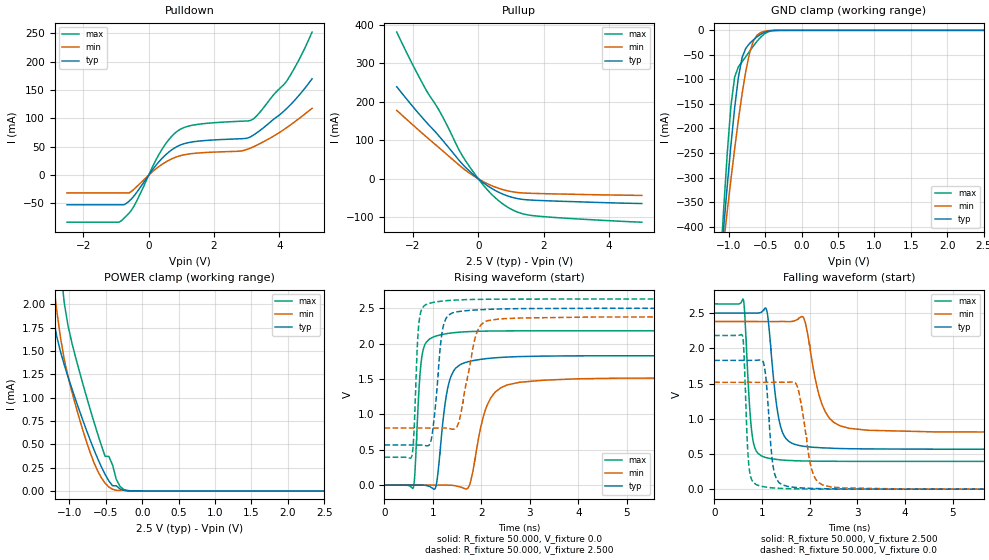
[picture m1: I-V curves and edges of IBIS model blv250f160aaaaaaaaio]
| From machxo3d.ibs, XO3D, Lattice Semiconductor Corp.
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|   Model blv250f160aaaaaaaaio
[Model] blv250f160aaaaaaaaio
Model_type I/O
Polarity   Non-Inverting
Enable   Active-Low
Vinl =  1.150V
Vinh =  1.350V
Vmeas =  1.250V
Cref =  3.000pF
Rref =  50.000
Vref =  1.250V
C_comp   4.200pF   3.800pF   7.500pF
[Temperature Range]   25.000   0.105k   -40.000
[Voltage Range]   2.500V   2.380V   2.630V
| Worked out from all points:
|   slope of the pulldown table from 0 to 0.375 V, typ, clamps not added: 13.6 ohm
|   slope of the pullup table from 0 to 0.375 V, typ, clamps not added: 16.3 ohm
|   GND clamp passes 1 mA (typ) near -0.43 V on its own axis
|   POWER clamp passes 1 mA (typ) near -0.92 V on its own axis
|   rising waveform, R_fixture 50.000, V_fixture 0.0: 20-80 % time 206ps typ, 326ps min, 111ps max; typ from 0 V to 1.83 V
|   rising waveform, R_fixture 50.000, V_fixture 2.500: 20-80 % time 152ps typ, 261ps min, 82.5ps max; typ from 0.567 V to 2.5 V
|   falling waveform, R_fixture 50.000, V_fixture 2.500: 20-80 % time 196ps typ, 321ps min, 119ps max; typ from 2.5 V to 0.567 V
|   falling waveform, R_fixture 50.000, V_fixture 0.0: 20-80 % time 127ps typ, 212ps min, 78.8ps max; typ from 1.83 V to 0 V
[Pulldown]
|Voltage   I(typ)   I(min)   I(max)
-2.5V     -52.31mA   -31.26mA   -82.98mA
-828mV    -52.31mA   -31.26mA   -79.94mA
-600mV    -45.86mA   -31.26mA   -66.93mA
-448mV    -36.56mA   -24.66mA   -54.4mA
160mV     12.89mA    8.306mA    19.88mA
464mV     32.88mA    21.18mA    50.69mA
996mV     53.81mA    34.73mA    81.8mA
1.528V    60.05mA    39.14mA    89.82mA
2.82V     64.22mA    42.56mA    95.13mA
3.2V      70.47mA    49.87mA    99.09mA
4.264V    119.9mA    85.51mA    169.5mA
5V        169.9mA    117.9mA    252.4mA
[Pullup]
|Voltage   I(typ)   I(min)   I(max)
-2.5V     238.9mA    177.6mA    380.6mA
-1.84V    170.7mA    127.3mA    268.1mA
-1.536V   141.5mA    104.8mA    221.1mA
-1.156V   106.1mA    77.3mA     170.6mA
-624mV    51.53mA    38.3mA     80.07mA
-472mV    36.72mA    27.5mA     57.26mA
136mV     -9.136mA   -6.562mA   -14.75mA
364mV     -22.46mA   -16.03mA   -36.5mA
668mV     -36.45mA   -25.77mA   -59.89mA
1.124V    -49.7mA    -34.48mA   -83.45mA
1.58V     -54.71mA   -37.23mA   -94.24mA
5V        -63.82mA   -42.81mA   -112.2mA
[GND_clamp]
|Voltage   I(typ)   I(min)   I(max)
-2.5V     -3.262A    -2.545A    -4.485A
-1.123V   -498.5mA   -505.1mA   -498.3mA
-1.072V   -406.1mA   -436mA     -369.4mA
-1.021V   -317.1mA   -368.7mA   -251mA
-970mV    -233.3mA   -303.5mA   -153.4mA
-919mV    -157.7mA   -241.1mA   -95.21mA
-868mV    -95.78mA   -182.7mA   -74.26mA
-817mV    -55.48mA   -129.4mA   -63.96mA
-715mV    -26.89mA   -46.57mA   -42.82mA
-562mV    -8.195mA   -4.484mA   -13.98mA
-358mV    -153.4uA   -68.26uA   -250.2uA
2.5V      0A         0A         0A
[POWER_clamp]
|Voltage   I(typ)   I(min)   I(max)
-2.5V     19.37mA    14.08mA    35.47mA
-1.274V   2.185mA    2.634mA    5.424mA
-1.223V   1.865mA    2.265mA    4.051mA
-1.172V   1.654mA    1.93mA     3.052mA
-1.07V    1.353mA    1.412mA    2.016mA
-968mV    1.104mA    1.071mA    1.597mA
-815mV    758.5uA    651.8uA    1.15mA
-509mV    176.7uA    82.75uA    370.5uA
-407mV    55.24uA    18.01uA    278.8uA
-305mV    21.57uA    6.5uA      49.89uA
-203mV    2.401uA    2.25uA     4.21uA
2.5V      0A         0A         3.059nA
[Ramp]
| variable   typ   min   max
dV/dt_r   1.097/0.206n   0.910/0.325n   1.309/0.110n
dV/dt_f   1.160/0.196n   0.944/0.320n   1.341/0.119n
R_load = 50.000
[Rising Waveform]
R_fixture= 50.000
V_fixture= 0.0
V_fixture_min= 0.0
V_fixture_max= 0.0
|time   V(typ)   V(min)   V(max)
0s        6.258nV    42.73nV    18.47nV
597ps     -200.6uV   920nV      -35.25mV
718ps     -428.8uV   920nV      1.422V
769ps     -516.5uV   920nV      1.805V
1.036ns   -57.26mV   -22.87uV   2.101V
1.3ns     1.356V     -654.9uV   2.144V
1.725ns   1.745V     -39mV      2.169V
2.119ns   1.789V     1.132V     2.177V
2.781ns   1.817V     1.453V     2.181V
20ns      1.829V     1.517V     2.182V
[Rising Waveform]
R_fixture= 50.000
V_fixture= 2.500
V_fixture_min= 2.380
V_fixture_max= 2.630
|time   V(typ)   V(min)   V(max)
0s        567.4mV    806.9mV    394.6mV
565ps     567.2mV    806.9mV    412.4mV
727ps     567mV      806.9mV    2.377V
951ps     604.4mV    806.7mV    2.574V
1.068ns   1.238V     806.2mV    2.591V
1.27ns    2.359V     806.8mV    2.607V
1.525ns   2.452V     871.4mV    2.618V
1.939ns   2.478V     2.213V     2.626V
2.376ns   2.49V      2.35V      2.629V
20ns      2.5V       2.38V      2.63V
[Falling Waveform]
R_fixture= 50.000
V_fixture= 2.500
V_fixture_min= 2.380
V_fixture_max= 2.630
|time   V(typ)   V(min)   V(max)
0s        2.5V       2.38V      2.63V
610ps     2.499V     2.38V      2.693V
801ps     2.5V       2.38V      738.5mV
1.084ns   2.57V      2.38V      448mV
1.192ns   1.947V     2.38V      432.3mV
1.508ns   714mV      2.379V     410mV
1.876ns   609.5mV    2.431V     399.7mV
2.253ns   587.2mV    1.214V     396.2mV
2.823ns   574.3mV    864.2mV    394.9mV
20ns      567.3mV    806.9mV    394.5mV
[Falling Waveform]
R_fixture= 50.000
V_fixture= 0.0
V_fixture_min= 0.0
V_fixture_max= 0.0
|time   V(typ)   V(min)   V(max)
0s        1.829V     1.517V     2.182V
594ps     1.828V     1.517V     2.177V
736ps     1.829V     1.517V     278.8mV
1.085ns   1.568V     1.517V     29.01mV
1.267ns   213.9mV    1.517V     15.96mV
1.649ns   28.04mV    1.523V     5.319mV
1.782ns   19.34mV    1.354V     3.815mV
2.078ns   10.17mV    205.1mV    1.609mV
2.445ns   5.144mV    31.58mV    507.2uV
20ns      -109.5nV   -67.12nV   -21.07nV
